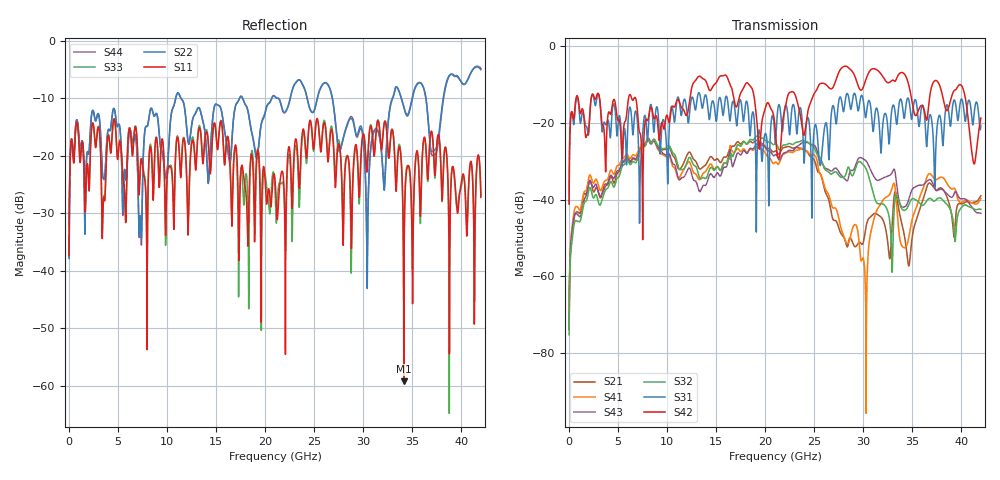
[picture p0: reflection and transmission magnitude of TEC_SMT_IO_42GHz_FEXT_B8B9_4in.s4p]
!! CHANNEL DESCRIPTION: Next Generation 28Gbps High Density SMT I/O Connector
!!  with 4" 5-6-5 Megatron 6 Stripline trace on host side and 1.25" 7-5-7 Megtron 6 Microstrip trace on plug side at 14GHz
!! HOST PCB DESCRIPTION: PCB thickness 2.86 mm, Nelco 4000-13SI (Dk 3.32, Df 0.010)
!!  23 Layer Board, 12 GND planes, 2 Layer route-out on Layers 10,12, 8 mil stub on vias
!!  Pairs on following layers
!!  Layer 10 - B8B9
!! CONNECTOR DESCRIPTION:  Next Generation 28Gbps High Density SMT I/O Connector
!! PLUG-IN CARD DESCRIPTION:  PCB thickness 1mm thick, Nelco 4000-13SI (Dk 3.32, Df 0.010)
!!  6 Layer Board, 4 GND planes, 0.35 x 1.4mm mating pads
!!  Micro-strip diff traces referenced to GND plane 3mils down, 2nd GND plane 15mils from top of board
!!  PCB GND planes are symmetric
!! MODEL DESCRIPTION: TE Connectivity S-parameter model produced from Macro-model
!! MODEL DATE: 9/25/2014 CR1a_GC1i, VR6&12_4
!! MODEL STATUS: Developmental
!! MODEL GEOMETRY: 2 Rows - Rows A, B. 3 pairs in each row, 6 total pairs
!! MODEL FREQUENCY RANGE: DC to 42 GHz in 10 MHz frequency steps
!! MODEL EDGE RATE LIMITATION: 11.90 ps (Using conservative 0.5/Fmax rule of thumb)
!! TIME-DOMAIN TRANSFORM CAUTIONS:
!! 1.) Do not simulate transient edge rates faster than the number listed above.  Edge
!!  rates faster than this number contain significant spectral content at frequencies
!!  above the model's highest frequency.
!! 2.) Even when simulating edge rates that are slower than the number listed above, be
!!  aware that the best time resolution possible with a direct iFFT is (1 / 2Fmax).
!!  As a result, time resolution is typically not adequate for most time-domain
!!  simulations unless tricks such as frequency-domain zero-padding and windowing are
!!  used to minimize leakage and aliasing.
!! 3.) Because the model has a uniform frequency step, a direct iFFT will result in an
!!  impulse that that has a time length given by either (1 / Fstep) or (1 / 2Fstep),
!!  depending on the transform being used.  Care has been taken in selecting the
!!  frequency step to ensure a settled impulse response for the model.  Therefore,
!!  convolution with the model's impulse response should present no issues.  However,
!!  if directly concatenating s-parameter models in the frequency domain a user must
!!  either interpolate necessary interim frequencies or complete impulse response
!!  zero-padding.  Impulse response zero-padding is more difficult, but more accurate.
!! PORT DEFINITIONS:
!! Port  1  ----->  Host, Bot Row  B8  B5  Module, Top Row  <-----  Port  2
!! Port  3  ----->  Host, Bot Row  B9  B6  Module, Top Row  <-----  Port  4
# Hz S MA R 50
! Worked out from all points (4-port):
!   4200 points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, 10 MHz to 42 GHz, reference 50 ohm
!   strongest paths, dB at 10 MHz, 10.51 GHz, 21.01 GHz, 31.51 GHz, 42 GHz:
!     S42: -41.1, -15.7, -21.2, -6.3, -18.7
!     S31: -41.2, -15.7, -24.6, -17.4, -20.6
!     S32: -75.4, -27.5, -25.5, -41.1, -42.6
!     S43: -73.8, -30.2, -28.3, -35.0, -43.6
!     S41: -72.5, -30.9, -30.3, -42.2, -39.7
!     S21: -74.0, -28.1, -27.3, -44.0, -39.0
!   lowest |S11| = -59.2 dB at 34.14 GHz (marker M1), VSWR 1.00, Z = 50 + j0.109 ohm
!   |S11| at or under -10 dB: start of sweep to end of sweep
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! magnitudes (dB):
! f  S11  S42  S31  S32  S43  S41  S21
! 10 MHz  -37.3  -41.1  -41.2  -75.4  -73.8  -72.5  -74.0
! 2.07 GHz  -25.6  -19.5  -20.0  -37.0  -35.2  -33.7  -35.2
! 8.07 GHz  -25.2  -19.0  -22.5  -24.3  -24.5  -24.1  -23.9
! 24.99 GHz  -18.5  -12.4  -21.9  -26.4  -25.7  -28.4  -29.6
! 30.41 GHz  -22.2  -7.7  -15.8  -32.7  -30.4  -59.3  -45.8
! 34.14 GHz  -59.2  -7.0  -18.5  -42.8  -42.0  -52.5  -48.6
! 42 GHz  -27.3  -18.7  -20.6  -42.6  -43.6  -39.7  -39.0
